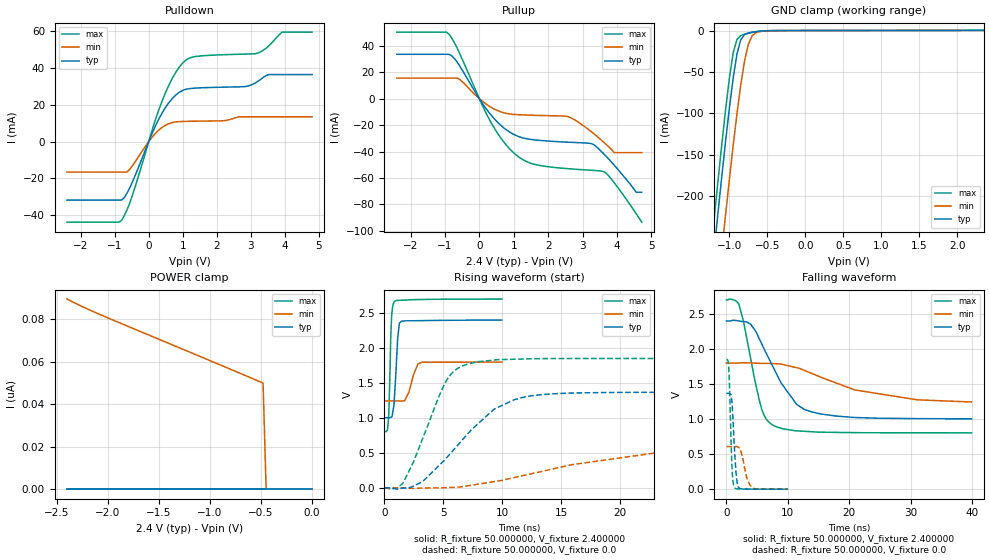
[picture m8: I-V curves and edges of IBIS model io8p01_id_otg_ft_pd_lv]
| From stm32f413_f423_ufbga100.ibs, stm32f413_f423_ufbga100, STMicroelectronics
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|   Model io8p01_id_otg_ft_pd_lv
[Model]  io8p01_id_otg_ft_pd_lv
Model_type I/O
Polarity   Non-Inverting
Enable   Active-Low
Vinl =   0.720000V
Vinh =   1.680000V
Vmeas =  1.200000V
Cref =   50.000000pF
Rref =   100.000000M
Vref =   0.0V
C_comp   2.229800pF   2.169700pF   2.325100pF
[Temperature Range]   25.000000   0.125000k   -40.000000
[Pullup Reference]   2.400000V   1.800000V   2.700000V
[Pulldown Reference]   0.0V   0.0V   0.0V
[POWER Clamp Reference]   2.400000V   1.800000V   2.700000V
[GND Clamp Reference]   0.0V   0.0V   0.0V
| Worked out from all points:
|   slope of the pulldown table from 0 to 0.36 V, typ, clamps not added: 25 ohm
|   slope of the pullup table from 0 to 0.36 V, typ, clamps not added: 27.7 ohm
|   GND clamp passes 1 mA (typ) near -0.62 V on its own axis
|   rising waveform, R_fixture 50.000000, V_fixture 2.400000: 20-80 % time 274ps typ, 609ps min, 184ps max; typ from 1 V to 2.4 V
|   rising waveform, R_fixture 50.000000, V_fixture 0.0: 20-80 % time 4.75ns typ, 12.1ns min, 2.63ns max; typ from 0 V to 1.37 V
|   falling waveform, R_fixture 50.000000, V_fixture 2.400000: 20-80 % time 5.33ns typ, 12.4ns min, 2.68ns max; typ from 2.4 V to 1 V
|   falling waveform, R_fixture 50.000000, V_fixture 0.0: 20-80 % time 523ps typ, 974ps min, 382ps max; typ from 1.37 V to 0 V
[Pulldown]
|Voltage   I(typ)   I(min)   I(max)
-2.4V     -31.73mA   -16.51mA   -43.74mA
-800mV    -31.73mA   -16.51mA   -42.87mA
-480mV    -21.97mA   -13.17mA   -29.2mA
80mV      3.629mA    1.966mA    5.013mA
480mV     18.15mA    8.737mA    26.01mA
800mV     25.37mA    10.71mA    37.77mA
1.12V     28.53mA    11.02mA    44.6mA
2.8V      29.83mA    13.48mA    47.51mA
3.2V      32.64mA    13.48mA    48.03mA
3.52V     36.41mA    13.48mA    51.82mA
3.92V     36.41mA    13.48mA    59.47mA
4.8V      36.41mA    13.48mA    59.47mA
[Pullup]
|Voltage   I(typ)   I(min)   I(max)
-2.4V     33.56mA    15.56mA    50.36mA
-960mV    33.56mA    15.56mA    50.36mA
-560mV    24.28mA    14.3mA     33.54mA
320mV     -11.75mA   -6.207mA   -17.08mA
960mV     -26.47mA   -11.82mA   -40.02mA
1.52V     -30.88mA   -12.51mA   -49.05mA
2.56V     -32.88mA   -13.48mA   -52.9mA
3.28V     -34.19mA   -25.52mA   -54.18mA
3.6V      -41.31mA   -32.62mA   -54.98mA
3.92V     -50.33mA   -40.8mA    -63.62mA
4.56V     -70.8mA    -40.8mA    -87.07mA
4.72V     -70.8mA    -40.8mA    -93.4mA
[GND_clamp]
|Voltage   I(typ)   I(min)   I(max)
-2.4V     -1.424A    -1.508A    -1.393A
-1.25V    -311.2mA   -401.9mA   -273.3mA
-1.2V     -265.4mA   -356.1mA   -227.2mA
-1.15V    -220.4mA   -310.8mA   -181.9mA
-1.1V     -176.3mA   -266.2mA   -137.9mA
-1.05V    -133.8mA   -222.5mA   -95.89mA
-950mV    -57.33mA   -138.9mA   -27.03mA
-900mV    -28.31mA   -100.4mA   -10.67mA
-850mV    -11.07mA   -65.56mA   -6.047mA
-750mV    -2.904mA   -16.55mA   -3.26mA
-600mV    -808.2uA   -1.212mA   -806.8uA
2.35V     242.6uA    152uA      283.9uA
[POWER_clamp]
|Voltage   I(typ)   I(min)   I(max)
-2.4V     0A         89.62nA    0A
-2.04V    0A         81.58nA    0A
-480mV    0A         50.01nA    0A
-450mV    0A         0A         0A
0V        0A         0A         0A
[Ramp]
| variable   typ   min   max
dV/dt_r  0.81972/4.74740n   0.38296/12.98931n   1.10814/2.62236n
dV/dt_f  0.83652/5.33582n   0.32454/13.33360n   1.13626/2.67745n
R_load = 50.000000
[Rising Waveform]
R_fixture= 50.000000
V_fixture= 2.400000
V_fixture_min= 1.800000
V_fixture_max= 2.700000
|time   V(typ)   V(min)   V(max)
0s        1.003V     1.242V     802.8mV
260.3ps   1.003V     1.242V     829mV
340.3ps   1.002V     1.242V     985.7mV
600.6ps   1.011V     1.242V     2.429V
860.9ps   1.335V     1.242V     2.662V
1.121ns   2.133V     1.242V     2.677V
1.381ns   2.372V     1.24V      2.679V
1.722ns   2.385V     1.25V      2.681V
3.203ns   2.388V     1.794V     2.69V
9.97ns    2.396V     1.796V     2.696V
[Rising Waveform]
R_fixture= 50.000000
V_fixture= 0.0
V_fixture_min= 0.0
V_fixture_max= 0.0
|time   V(typ)   V(min)   V(max)
0s        178uV      73.93uV    445.1uV
1.602ns   -2.678mV   -101.3uV   77.5mV
3.283ns   96.81mV    -688.3uV   721.7mV
5.125ns   401.2mV    3.286mV    1.491V
5.926ns   553.2mV    8.881mV    1.669V
7.047ns   766mV      29.21mV    1.767V
9.369ns   1.129V     91.25mV    1.826V
13.05ns   1.326V     223.9mV    1.845V
24.82ns   1.365V     541mV      1.848V
39.88ns   1.366V     606.5mV    1.847V
[Falling Waveform]
R_fixture= 50.000000
V_fixture= 2.400000
V_fixture_min= 1.800000
V_fixture_max= 2.700000
|time   V(typ)   V(min)   V(max)
0s        2.396V     1.796V     2.696V
2.002ns   2.395V     1.797V     2.639V
2.803ns   2.387V     1.801V     2.376V
3.924ns   2.351V     1.798V     1.87V
5.766ns   2.065V     1.792V     1.132V
7.608ns   1.736V     1.788V     909.9mV
11.37ns   1.214V     1.731V     831.2mV
13.93ns   1.1V       1.647V     817.7mV
20.9ns    1.021V     1.414V     805.4mV
39.88ns   1.003V     1.242V     802.8mV
[Falling Waveform]
R_fixture= 50.000000
V_fixture= 0.0
V_fixture_min= 0.0
V_fixture_max= 0.0
|time   V(typ)   V(min)   V(max)
0s        1.366V     606.5mV    1.847V
380.4ps   1.366V     606.5mV    1.715V
480.5ps   1.366V     606.5mV    1.517V
880.9ps   1.252V     606.3mV    357.4mV
1.061ns   998.8mV    606mV      112.1mV
1.261ns   651.3mV    605.9mV    33.58mV
1.702ns   116.4mV    608mV      4.921mV
2.062ns   17.35mV    591mV      2.714mV
3.864ns   959.2uV    52.29mV    1.312mV
9.97ns    178uV      73.93uV    445.1uV
